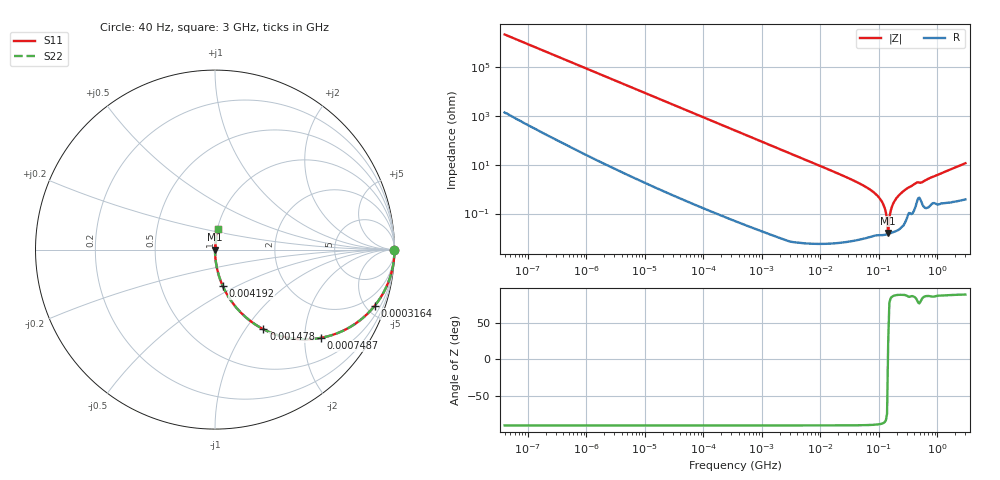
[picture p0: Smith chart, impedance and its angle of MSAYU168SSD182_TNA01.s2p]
! MSAYU168SSD182_TNA01  S-PARAMETER MODEL  ( General Type )
! Model Generated by TAIYO YUDEN Corporation (http://www.ty-top.com)
! Version 2.0
! TAIYO YUDEN Control No. 030711
! Copyright(c) 2003 TAIYO YUDEN CO.,LTD. All Rights Reserved.
! Product Description (link to TY-COMPAS)
! https://ds.yuden.co.jp/TYCOMPAS/or/detail?pn=MSAYU168SSD182KTNA01&u=M
! Products Name : Multilayer Ceramic Capacitors
! Characteristics :
!  Capacitance : 1800 pF , Rated Voltage : 50V
!  Case Size : 1.6 x 0.8 / 0.063 x 0.031 [mm/inch] , Thickness : 0.8 / 0.031 [mm/inch]
!  (Conditions: Temperature = 25 degC , DC Bias Current/Voltage = 0A / 0V)
! External Node Assignments :
!  1  o---| |---o  2
! GND o---------o GND
! Frequency Range : 40Hz  -  3GHz  [ 401 STEP ]
# MHz S RI R 50
! Freq[MHz].  S11 Real  S11 Imag  S21 Real  S21 Imag  S12 Real  S12 Imag  S22 Real  S22 Imag
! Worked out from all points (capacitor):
!   401 points, 40 Hz to 3 GHz, reference 50 ohm
!   read as one part in series: C = 1.77 nF near 44 Hz
!   lowest |Z| = 16.1 mohm at 143.9 MHz (marker M1)
!   series resonance near 143.1 MHz, so ESL is about 700 pH
!   S11 on the Smith chart (normalised r, x): 40 Hz: open; 316.4 kHz: 1.00, -5.67; 748.7 kHz: 1.00, -2.40; 1.478 MHz: 1.00, -1.21; 4.192 MHz: 1.00, -0.43; 3 GHz: 1.01, +0.23
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4e-05  1 -4.46e-05  3e-08 4.46e-05  3e-08 4.46e-05  1 -4.46e-05
9.5e-05  1 -0.000106  6.3e-08 0.000106  6.3e-08 0.000106  1 -0.000106
0.000834  1 -0.000929  1.13e-06 0.000929  1.13e-06 0.000929  1 -0.000929
0.017386  0.9996 -0.0194  0.000379 0.0194  0.000379 0.0194  0.9996 -0.0194
0.093035  0.9894 -0.1025  0.0106 0.1025  0.0106 0.1025  0.9894 -0.1025
0.316385  0.8894 -0.3135  0.1106 0.3135  0.1106 0.3135  0.8894 -0.3135
0.362475  0.8597 -0.3472  0.1403 0.3472  0.1403 0.3472  0.8597 -0.3472
0.748653  0.5897 -0.4918  0.4103 0.4918  0.4103 0.4918  0.5897 -0.4918
1.477731  0.2695 -0.4436  0.7305 0.4436  0.7305 0.4436  0.2695 -0.4436
4.191906  0.0438 -0.2045  0.9562 0.2045  0.9562 0.2045  0.0438 -0.2045
7.222098  0.0152 -0.1221  0.9848 0.1221  0.9848 0.1221  0.0152 -0.1221
76.28187  0.000187 -0.00842  0.9998 0.00842  0.9998 0.00842  0.000187 -0.00842
109.6283  0.000142 -0.00338  0.9999 0.00338  0.9999 0.00338  0.000142 -0.00338
120.0322  0.000137 -0.00222  0.9999 0.00222  0.9999 0.00222  0.000137 -0.00222
131.4235  0.000139 -0.00109  0.9999 0.00109  0.9999 0.00109  0.000139 -0.00109
143.8959  0.000146 6.61e-05  0.9999 -6.61e-05  0.9999 -6.61e-05  0.000146 6.61e-05
150.5692  0.000152 0.000647  0.9998 -0.000647  0.9998 -0.000647  0.000152 0.000647
172.504  0.000175 0.00238  0.9998 -0.00238  0.9998 -0.00238  0.000175 0.00238
188.875  0.000198 0.00357  0.9998 -0.00357  0.9998 -0.00357  0.000198 0.00357
284.0294  0.000561 0.00969  0.9994 -0.00969  0.9994 -0.00969  0.000561 0.00969
427.1222  0.00244 0.0176  0.9976 -0.0176  0.9976 -0.0176  0.00244 0.0176
3000  0.017 0.1141  0.983 -0.1141  0.983 -0.1141  0.017 0.1141
